(* 	
	Program Name: 	ACS_MOVE_INDEXED
	Purpose:		Copy Index Move to ACS Drive Output Register
	When Executed:	Primes Output Registers for an Indexed Move to be executed upon Start Motion command
*)
PROGRAM ACS_MOVE_INDEXED
VAR_IN_OUT
	Axis:ACS_DRIVE_TYPE;
END_VAR

VAR_INPUT
	// Executes profile at given index table (defined in TMI)
	IndexPosition: USINT;
END_VAR

VAR
	_moveType:UDINT := ACS_MOTION_TYPES.FORCE;
END_VAR

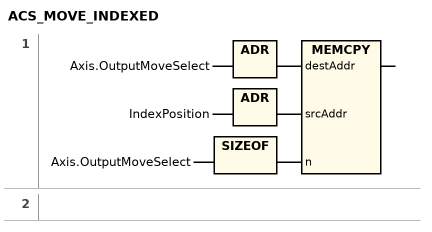
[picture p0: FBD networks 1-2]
// NETWORK 1
MEMCPY(destAddr := ADR(Axis.OutputMoveSelect), srcAddr := ADR(IndexPosition), n := SIZEOF(Axis.OutputMoveSelect));

// NETWORK 2

END_PROGRAM
